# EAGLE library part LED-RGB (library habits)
LED-RGB 6 pin RGB LED (no common connector) Packages: PLCC-6 LED-TRICOLOR-5050 - No built-in IC SparkFun Products: Digital Sandbox LED- SMD RGB
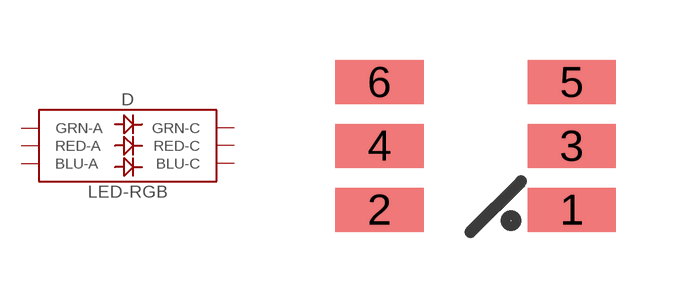
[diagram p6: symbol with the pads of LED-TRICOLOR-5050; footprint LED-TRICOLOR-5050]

Designator prefix D

## LED-RGBBRG (PROD_ID: DIO-16048)  [LED-TRICOLOR-5050]
1  BLU-C
2  BLU-A
3  RED-C
4  RED-A
5  GRN-C
6  GRN-A

## Footprint LED-TRICOLOR-5050 (pad centres in mm)
5050 SMD RGB LED Specifications: Pin count: 6 Pin pitch: 0.6mm Area: 5.0mm x 5.mm Thickness: 2.6mm Datasheet referenced for footprint: 5060BRG4 Example device(s): LED-RGB
smd 2.2 x 1.1: 1 2.781,-1.6; 2 -2.019,-1.6; 3 2.781,0; 4 -2.019,0; 5 2.781,1.6; 6 -2.019,1.6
